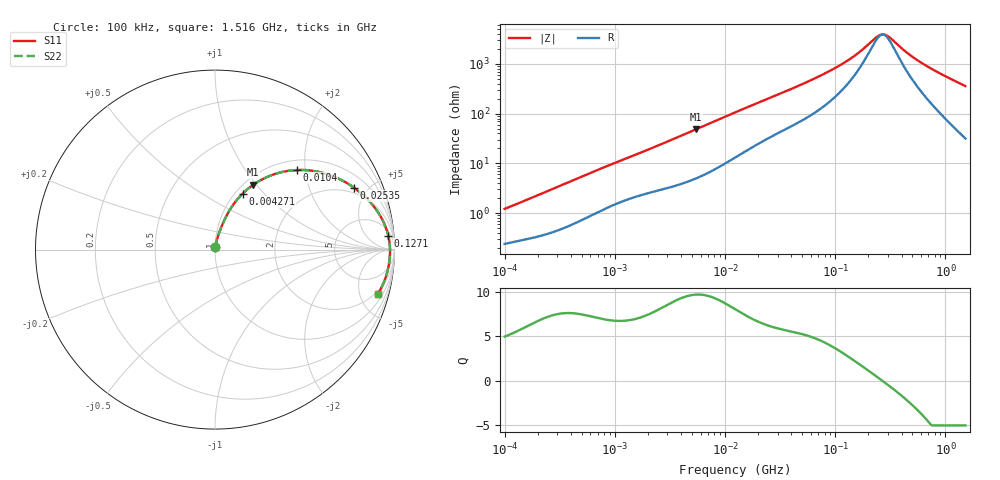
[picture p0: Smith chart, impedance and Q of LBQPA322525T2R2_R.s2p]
! LBQPA322525T2R2_R  S-PARAMETER MODEL  ( General Type )
! Model Generated by TAIYO YUDEN Corporation (http://www.ty-top.com)
! Version 1.0
! TAIYO YUDEN Control No. 191025NI43SB-FBB
! Copyright(c) 2019 TAIYO YUDEN CO.,LTD. All Rights Reserved.
! Product Description (link to TY-COMPAS)
! https://ds.yuden.co.jp/TYCOMPAS/or/detail?pn=LBQPA322525T2R2MR&u=M
! Products Name : Inductors
! Characteristics :
!  Inductance : 2.2 uH , SRF(min) : 190 MHz , DC Resistance(max) : 0.104 Ohm
!  Rated Current : Saturation :2000 mA , Temp Rise : 930 mA (20 degC)
!  Case Size : 3.2 x 2.5 / 0.126 x 0.098 [mm/inch] , Thickness : 2.5 / 0.098 [mm/inch]
!  (Conditions: Temperature = 25 degC , DC Bias Current/Voltage = 0A / 0V)
! External Node Assignments :
!  1  o---GGG---o  2
! GND o---------o GND
! Frequency Range : 0.1MHz  -  1516.370183MHz  [ 402 STEP ]
# MHz S RI R 50
! Freq[MHz].  S11 Real  S11 Imag  S21 Real  S21 Imag  S12 Real  S12 Imag  S22 Real  S22 Imag
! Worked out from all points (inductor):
!   401 points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, 100 kHz to 1.516 GHz, reference 50 ohm
!   read as one part in series: L = 1.86 uH near 104.9 kHz
!   highest Q = 9.7 at 5.433 MHz (marker M1), where L = 1.41 uH
!   self-resonance near 269.1 MHz
!   S11 on the Smith chart (normalised r, x): 100 kHz: 1.00, +0.02; 4.271 MHz: 1.08, +0.76; 10.4 MHz: 1.21, +1.80; 25.35 MHz: 1.66, +4.08; 127.1 MHz: 9, +22; 1.516 GHz: 1.63, -7.17
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0.1  0.00254 0.0119  0.9975 -0.0119  0.9975 -0.0119  0.00254 0.0119
0.501516  0.0101 0.0532  0.9899 -0.0532  0.9899 -0.0532  0.0101 0.0532
1.221826  0.0311 0.1148  0.9689 -0.1148  0.9689 -0.1148  0.0311 0.1148
2.515184  0.0748 0.2082  0.9252 -0.2082  0.9252 -0.2082  0.0748 0.2082
4.270847  0.1532 0.3111  0.8468 -0.3111  0.8468 -0.3111  0.1532 0.3111
5.432931  0.2132 0.3613  0.7868 -0.3613  0.7868 -0.3613  0.2132 0.3613
7.794969  0.3365 0.4222  0.6635 -0.4222  0.6635 -0.4222  0.3365 0.4222
10.40492  0.4555 0.4433  0.5445 -0.4433  0.5445 -0.4433  0.4555 0.4433
12.61405  0.5367 0.44  0.4633 -0.44  0.4633 -0.44  0.5367 0.44
25.34913  0.776 0.3437  0.224 -0.3437  0.224 -0.3437  0.776 0.3437
39.09302  0.8672 0.2614  0.1328 -0.2614  0.1328 -0.2614  0.8672 0.2614
61.75718  0.9257 0.1796  0.0743 -0.1796  0.0743 -0.1796  0.9257 0.1796
90.76527  0.9528 0.1207  0.0472 -0.1207  0.0472 -0.1207  0.9528 0.1207
127.13  0.9656 0.0775  0.0344 -0.0775  0.0344 -0.0775  0.9656 0.0775
165.6609  0.9712 0.0481  0.0288 -0.0481  0.0288 -0.0481  0.9712 0.0481
249.4045  0.975 0.00732  0.025 -0.00732  0.025 -0.00732  0.975 0.00732
274.6074  0.9752 -0.00195  0.0248 0.00195  0.0248 0.00195  0.9752 -0.00195
309.7222  0.9752 -0.0136  0.0248 0.0136  0.0248 0.0136  0.9752 -0.0136
444.378  0.9732 -0.0503  0.0268 0.0503  0.0268 0.0503  0.9732 -0.0503
593.1667  0.9687 -0.0839  0.0313 0.0839  0.0313 0.0839  0.9687 -0.0839
937.0548  0.9523 -0.1506  0.0477 0.1506  0.0477 0.1506  0.9523 -0.1506
1516.37  0.9097 -0.2458  0.0903 0.2458  0.0903 0.2458  0.9097 -0.2458
